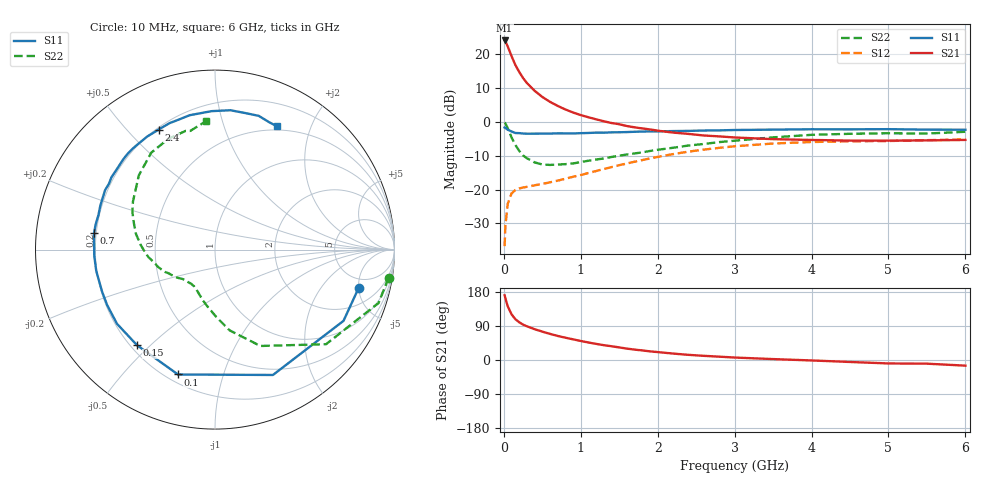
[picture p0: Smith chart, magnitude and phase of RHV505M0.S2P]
! SIEMENS Small Signal Semiconductors
! BFR106
! Si NPN RF Bipolar Junction Transistor in SOT23
! VCE = 0.5 V  IC = 5 mA
! Common Emitter S-Parameters:  August  1996
# GHz  S  MA  R  50
!  f  S11  S21  S12  S22
! GHz  MAG  ANG  MAG  ANG  MAG  ANG  MAG  ANG
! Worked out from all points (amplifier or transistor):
!   36 points, 10 MHz to 6 GHz, reference 50 ohm
!   highest |S21| = 24.1 dB at 10 MHz (marker M1)
!   |S21| within 3 dB of that: start of sweep to 71.94 MHz
!   unconditionally stable (mu >= 1): 563.5 MHz to end of sweep
!   at 250 MHz: K = 0.54, MSG = 16.2 dB, |S12| = -19.4 dB
!   at 1.4 GHz: K = 1.22, MAG = 3.7 dB, |S12| = -13.3 dB
!   at 6 GHz: K = 1.03, MAG = -1.2 dB, |S12| = -5.1 dB
!   S11 on the Smith chart (normalised r, x): 10 MHz: 3.68, -5.01; 100 MHz: 0.24, -0.72; 150 MHz: 0.23, -0.46; 700 MHz: 0.19, +0.07; 2.4 GHz: 0.21, +0.61; 6 GHz: 0.46, +1.53
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0.01  0.8285 -14.9  16.06 170.8  0.0146 83.2  0.98 -9.2
0.02  0.8187 -29.0  15.63 163.2  0.0289 75.1  0.9584 -18.1
0.05  0.7695 -65.2  13.14 142.0  0.0616 57.4  0.813 -40.4
0.1  0.7257 -106.5  9.447 120.5  0.0879 40.7  0.5934 -64.8
0.15  0.6874 -129.2  6.948 107.6  0.0987 32.8  0.4574 -79.7
0.2  0.6849 -142.9  5.496 99.6  0.104 30.0  0.3747 -89.0
0.25  0.6757 -152.8  4.468 93.3  0.1074 28.6  0.3203 -97.4
0.3  0.6713 -159.6  3.773 88.9  0.1101 28.5  0.2914 -103.3
0.4  0.6722 -169.8  2.898 81.3  0.1159 29.7  0.2529 -112.5
0.5  0.6735 -176.8  2.348 74.9  0.1215 32.0  0.2356 -119.6
0.6  0.675 176.9  1.987 68.9  0.1284 34.5  0.2321 -125.0
0.7  0.6799 172.1  1.732 63.5  0.1358 37.0  0.2351 -129.9
0.9  0.6773 163.5  1.383 54.5  0.1548 41.1  0.244 -138.0
1.1  0.6889 155.3  1.176 46.2  0.1762 44.1  0.2678 -145.3
1.3  0.6954 148.2  1.025 39.1  0.2018 45.7  0.2891 -152.7
1.6  0.7103 138.6  0.871 30.0  0.2441 45.9  0.3312 -163.0
2.2  0.7345 120.9  0.698 17.0  0.3356 40.5  0.4162 176.1
2.4  0.7387 115.2  0.667 13.6  0.3647 37.5  0.4492 168.7
3.5  0.7716 91.4  0.558 2.4  0.481 19.0  0.5928 135.7
4.5  0.7793 77.3  0.531 -5.2  0.5172 3.9  0.6697 112.8
5.5  0.7713 67.0  0.535 -9.7  0.5391 -4.7  0.6754 101.8
6  0.7689 63.2  0.543 -14.9  0.5539 -11.1  0.7171 94.0
